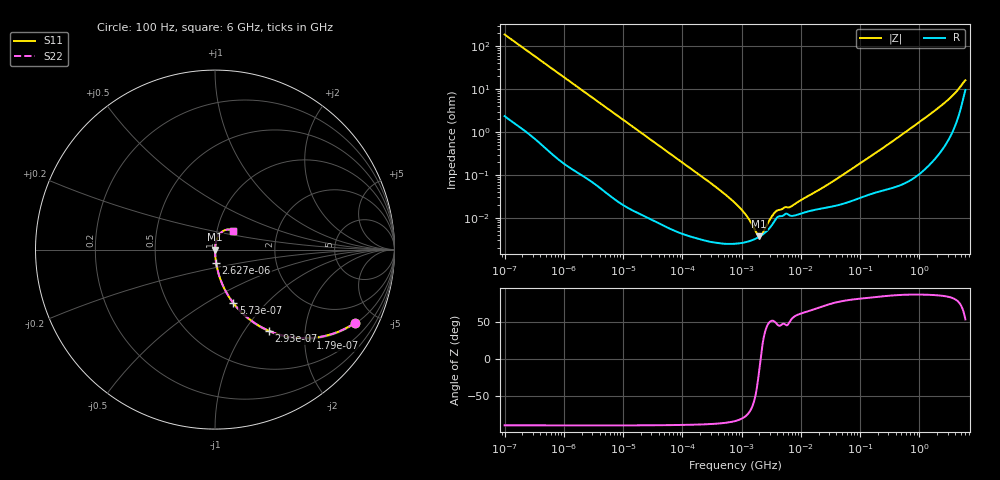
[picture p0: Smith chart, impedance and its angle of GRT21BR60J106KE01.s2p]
!Murata Part Number: GRT21BR60J106KE01
!These Parameters are Measured in Series Mode Connection
!Data Generated on Jun 19, 2026
!  o--ll--o
!Port1  Port2
!  o------o
!Operation Temp=25[degC], DC Bias Voltage=0[V]
!Freq. Start=100[Hz] Stop=6[GHz] 401[Steps]
# Hz S RI R 50
!Freq.(Hz) S11(Real) S11(Imag) S21(Real) S21(Imag) S12(Real) S12(Imag) S22(Real) S22(Imag)
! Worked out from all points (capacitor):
!   401 points, 100 Hz to 6 GHz, reference 50 ohm
!   read as one part in series: C = 8.4 uF near 109 Hz
!   lowest |Z| = 3.77 mohm at 1.983 MHz (marker M1)
!   series resonance near 2.091 MHz, so ESL is about 690 pH
!   S11 on the Smith chart (normalised r, x): 100 Hz: 1.05, -3.78; 179 Hz: 1.03, -2.12; 293 Hz: 1.02, -1.30; 573 Hz: 1.01, -0.67; 2.627 kHz: 1.00, -0.15; 6 GHz: 1.19, +0.26
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100  0.7782 -0.4092  0.2218 0.4092  0.2218 0.4092  0.7782 -0.4092
179  0.5288 -0.493  0.4712 0.493  0.4712 0.493  0.5288 -0.493
293  0.2996 -0.4521  0.7004 0.4521  0.7004 0.4521  0.2996 -0.4521
573  0.1029 -0.2986  0.8971 0.2986  0.8971 0.2986  0.1029 -0.2986
981  0.0386 -0.1878  0.9614 0.1878  0.9614 0.1878  0.0386 -0.1878
2008  0.0101 -0.0949  0.9899 0.0949  0.9899 0.0949  0.0101 -0.0949
2627  0.00614 -0.073  0.9939 0.073  0.9939 0.073  0.00614 -0.073
7695  0.000892 -0.0252  0.9991 0.0252  0.9991 0.0252  0.000892 -0.0252
40335  9.86e-05 -0.00487  0.9999 0.00487  0.9999 0.00487  9.86e-05 -0.00487
316350  2.77e-05 -0.000616  1 0.000616  1 0.000616  2.77e-05 -0.000616
774597  2.51e-05 -0.000223  1 0.000223  1 0.000223  2.51e-05 -0.000223
1325623  2.85e-05 -9e-05  1 9e-05  1 9e-05  2.85e-05 -9e-05
1983483  3.63e-05 -1.01e-05  1 1.01e-05  1 1.01e-05  3.63e-05 -1.01e-05
2967816  5.78e-05 6.77e-05  0.9999 -6.77e-05  0.9999 -6.77e-05  5.78e-05 6.77e-05
4060267  0.000105 0.000108  0.9999 -0.000108  0.9999 -0.000108  0.000105 0.000108
6948629  0.000111 0.00015  0.9999 -0.00015  0.9999 -0.00015  0.000111 0.00015
1.555665e7  0.00015 0.000334  0.9999 -0.000334  0.9999 -0.000334  0.00015 0.000334
3.80911e7  0.000192 0.000748  0.9998 -0.000748  0.9998 -0.000748  0.000192 0.000748
3.124326e8  0.000506 0.0054  0.9995 -0.0054  0.9995 -0.0054  0.000506 0.0054
2.34314e9  0.00528 0.041  0.9947 -0.041  0.9947 -0.041  0.00528 0.041
4.193612e9  0.0229 0.0822  0.9771 -0.0822  0.9771 -0.0822  0.0229 0.0822
6e9  0.1005 0.1055  0.8995 -0.1055  0.8995 -0.1055  0.1005 0.1055
